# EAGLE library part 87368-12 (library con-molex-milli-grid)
RECEPTACAL
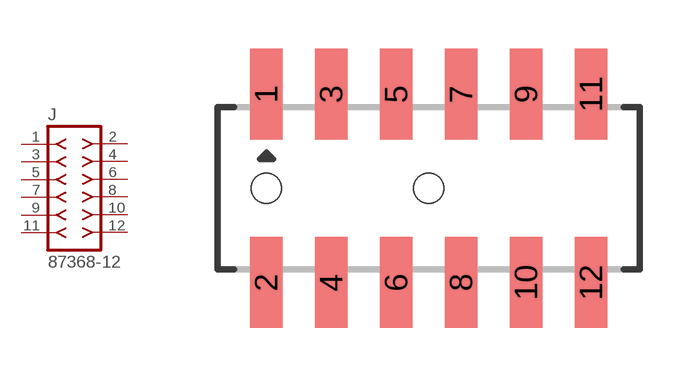
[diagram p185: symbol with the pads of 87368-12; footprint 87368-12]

Designator prefix J

## 87368-12  [87368-12]
1  1  pas
2  2  pas
3  3  pas
4  4  pas
5  5  pas
6  6  pas
7  7  pas
8  8  pas
9  9  pas
10  10  pas
11  11  pas
12  12  pas

## Footprint 87368-12 (pad centres in mm)
RECEPTACAL SMD Dual Row, Side Entry
smd 1 x 2.8: 1 -5,2.9; 2 -5,-2.9; 3 -3,2.9; 4 -3,-2.9; 5 -1,2.9; 6 -1,-2.9; 7 1,2.9; 8 1,-2.9; 9 3,2.9; 10 3,-2.9; 11 5,2.9; 12 5,-2.9
hole 0.914 at -5,0
hole 0.914 at 0,0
